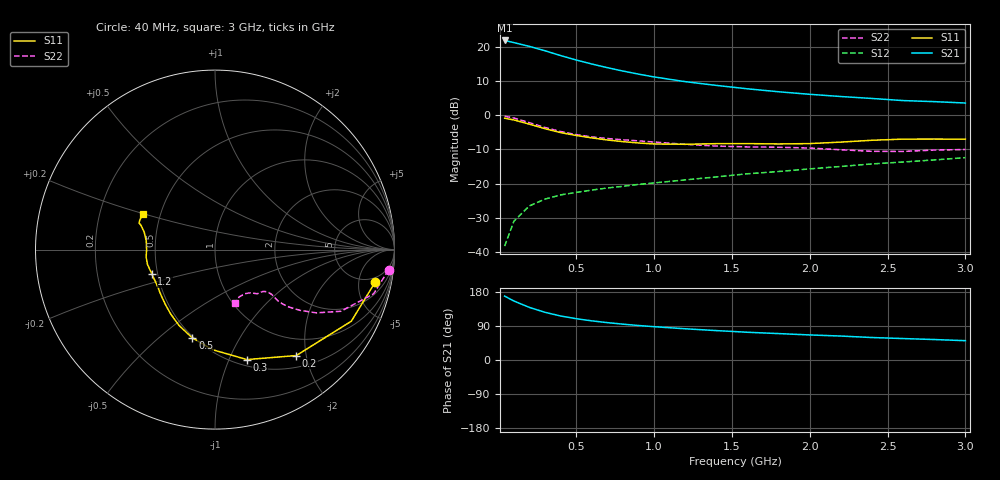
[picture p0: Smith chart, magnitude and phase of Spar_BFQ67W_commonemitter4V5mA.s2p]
! Filename:  BFQ67WB.S2P  Version:  4.0
! NXP part #: BFQ67W  Date: Jun 1994
! Bias condition: Vce=4V, Ic=5mA
#  MHz  S  MA  R  50
! Freq  S11  S21  S12  S22  !GUM [dB]
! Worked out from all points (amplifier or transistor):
!   21 points, 40 MHz to 3 GHz, reference 50 ohm
!   highest |S21| = 22.0 dB at 40 MHz (marker M1)
!   |S21| within 3 dB of that: start of sweep to 297 MHz
!   unconditionally stable (mu >= 1): 994.7 MHz to end of sweep
!   at 300 MHz: K = 0.45, MSG = 21.8 dB, |S12| = -24.6 dB
!   at 1 GHz: K = 1.00, MAG = 15.2 dB, |S12| = -19.8 dB
!   at 3 GHz: K = 1.06, MAG = 6.6 dB, |S12| = -12.4 dB
!   lowest NFmin = 1.50 dB at 1 GHz
!   S11 on the Smith chart (normalised r, x): 40 MHz: 3.80, -8.08; 200 MHz: 0.69, -1.82; 300 MHz: 0.56, -1.17; 500 MHz: 0.49, -0.65; 1.2 GHz: 0.46, -0.15; 3 GHz: 0.40, +0.20
40  0.91 -11.6  12.65 168.6  0.012 82.7  0.974 -6.7
100  0.858 -27.7  11.76 155.6  0.028 73.0  0.917 -15.6
200  0.744 -52.5  10.34 138.7  0.047 61.1  0.781 -26.1
300  0.638 -73.8  8.913 125.8  0.059 55.4  0.665 -32.0
400  0.559 -91.0  7.578 116.1  0.068 52.5  0.581 -35.6
500  0.508 -104.4  6.529 109.0  0.074 51.6  0.522 -37.8
600  0.468 -115.3  5.701 103.3  0.08 52.0  0.484 -38.8
700  0.436 -124.4  5.035 98.6  0.086 53.0  0.458 -39.2
800  0.412 -132.2  4.494 94.6  0.091 54.3  0.439 -39.0
900  0.394 -139.6  4.05 91.0  0.097 55.6  0.423 -38.7
1000  0.381 -146.6  3.683 87.9  0.102 56.9  0.407 -38.3
1200  0.377 -158.9  3.138 82.4  0.113 59.4  0.376 -38.7
1400  0.385 -167.5  2.764 77.6  0.125 61.7  0.355 -41.0
1600  0.386 -173.8  2.463 73.2  0.139 63.2  0.345 -44.3
1800  0.381 -179.8  2.229 69.7  0.15 65.2  0.341 -46.2
2000  0.386 172.8  2.045 66.1  0.164 66.7  0.332 -47.5
2200  0.406 166.2  1.897 63.2  0.178 68.3  0.313 -50.0
2400  0.432 162.1  1.777 59.3  0.194 69.2  0.297 -55.8
2600  0.449 160.6  1.654 56.6  0.207 69.4  0.296 -62.9
2800  0.45 158.3  1.596 54.0  0.222 70.6  0.31 -67.4
3000  0.448 153.7  1.523 51.0  0.24 71.0  0.316 -69.7
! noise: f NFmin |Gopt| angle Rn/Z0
1000  1.5  0.308  74  0.277
